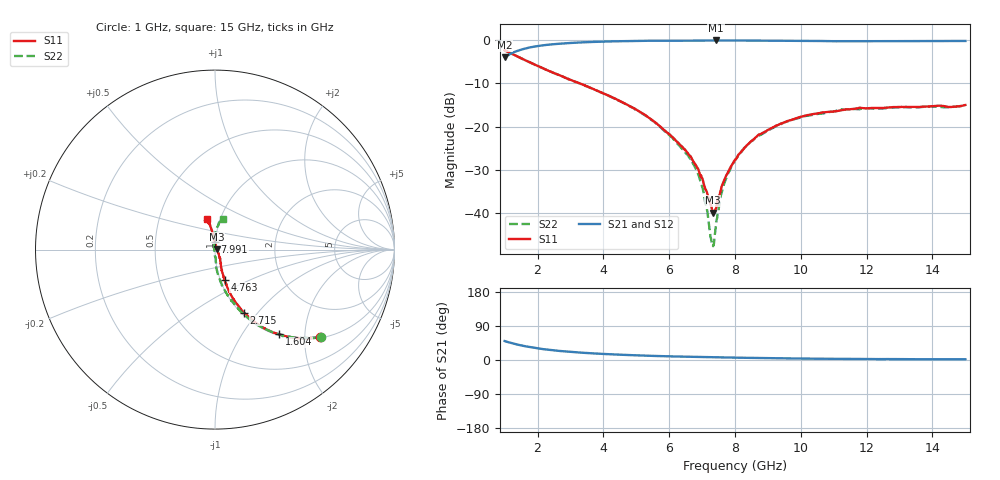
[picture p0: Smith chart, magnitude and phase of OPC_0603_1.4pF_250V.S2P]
! FILE NAME
! DATE 08/21/2012  09:54
! CORRECTED  DATA
# GHz  S  MA  R  50.00
!  FREQ  S11M  S11A  S21M  S21A  S12M  S12A  S22M  S22A
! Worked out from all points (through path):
!   1601 points, 1 GHz to 15 GHz, reference 50 ohm
!   highest |S21| = -0.06 dB at 7.423 GHz (marker M1); lowest = -3.9 dB at 1 GHz (marker M2)
!   group delay of S21, straight-line fit = 6.24 ps
!   lowest |S11| = -39.9 dB at 7.326 GHz (marker M3), VSWR 1.02, Z = 51 + j0.174 ohm
!   |S11| at or under -10 dB: 3.29 GHz to end of sweep
!   |S22| runs from -47.7 to -2.3 dB; largest |S21 - S12| = 0.0087
!   S11 on the Smith chart (normalised r, x): 1 GHz: 1.02, -2.39; 1.604 GHz: 1.02, -1.48; 2.715 GHz: 1.03, -0.85; 4.763 GHz: 1.05, -0.36; 7.991 GHz: 1.00, +0.08; 15 GHz: 0.87, +0.31
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1  0.7633 -39.7  0.6356 50.1  0.6354 49.9  0.7633 -39.5
1.60375  0.5918 -52.9  0.796 36.6  0.7961 36.6  0.5917 -52.9
2.715  0.3869 -65.2  0.9129 23.6  0.913 23.5  0.3854 -66.4
3.33625  0.3106 -68.9  0.9423 19.4  0.9416 19.3  0.3092 -71.4
4.7625  0.1758 -72.4  0.9776 13.1  0.9775 13.1  0.1754 -80.5
5.6725  0.1042 -71.0  0.9868 10.4  0.9866 10.4  0.1029 -85.5
6.48625  0.05379 -59.4  0.9858 8.8  0.9846 8.8  0.05 -86.1
6.81875  0.03521 -52.4  0.9886 8.3  0.9888 8.3  0.03187 -92.7
7.02  0.02417 -44.0  0.9907 8.0  0.99 8.0  0.01928 -100.1
7.11625  0.01853 -33.9  0.9906 7.8  0.9901 7.8  0.01255 -106.0
7.265  0.01256 -9.9  0.9916 7.5  0.9914 7.5  0.005208 -140.1
7.32625  0.01014 9.7  0.9924 7.4  0.9919 7.4  0.004295 173.8
7.4225  0.01138 44.6  0.9927 7.2  0.9911 7.2  0.007393 132.7
7.51  0.01566 59.9  0.9917 7.1  0.9914 7.1  0.0116 119.2
7.6325  0.02207 73.8  0.9922 6.9  0.9914 6.8  0.01925 109.9
7.99125  0.04081 89.6  0.9919 6.3  0.9912 6.3  0.03982 99.2
8  0.04119 89.1  0.992 6.2  0.9908 6.2  0.0405 99.5
8.735  0.08128 96.4  0.9896 5.3  0.989 5.3  0.07889 90.3
9.51375  0.1127 99.7  0.9858 4.4  0.9853 4.3  0.1118 86.6
10.33625  0.1387 101.2  0.9807 3.5  0.9799 3.5  0.136 82.2
12.6725  0.1663 108.4  0.9699 2.5  0.9698 2.4  0.1643 77.5
15  0.178 104.0  0.9794 2.0  0.979 2.0  0.175 75.5
